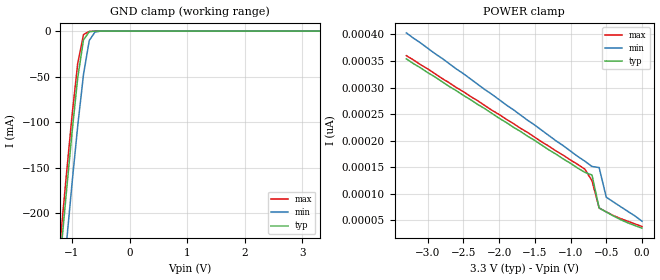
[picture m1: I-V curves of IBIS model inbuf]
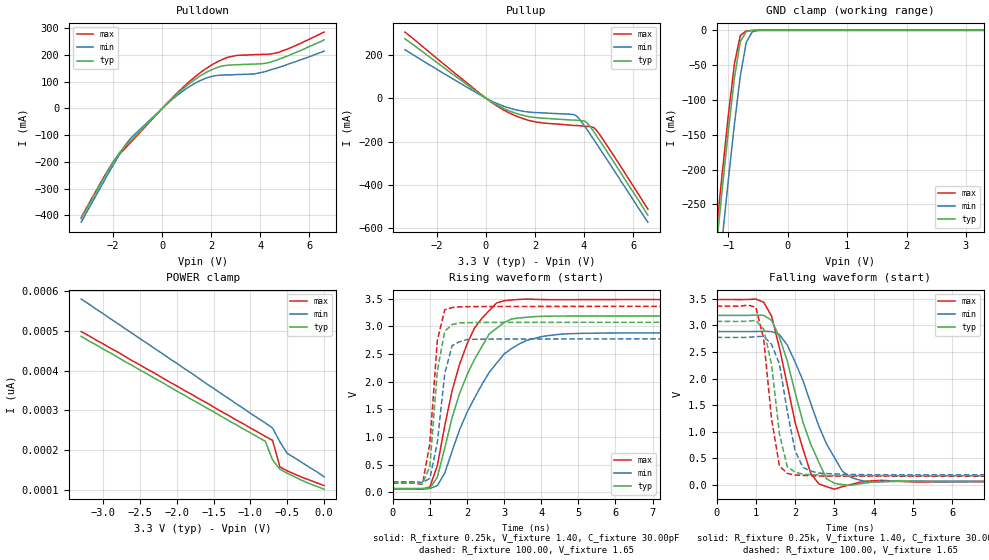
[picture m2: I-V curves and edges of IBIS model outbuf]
| IBIS file 163827.ibs created by s2ibis2 version 1.1
| North Carolina State University Electronics Research Laboratory  1995
[IBIS ver]   2.1
[File name]   163827.ibs
[File Rev]   1.0
[Date]   06/13/01
[Source]   Integrated Device Technology, Inc.
[Notes]   1.Temperatures: typ=25C, min=100C, max=0C 2.RRmp rates based
   on 50 ohm load.
[Disclaimer] Integrated Device Technology, Inc. ("IDT") hereby grants the
   user of this IBIS model a non-exclusive, nontransferable
   license to use this IBIS model under the following terms. The
   user is granted this license only to use the IBIS model and is
   not granted rights to sell, copy (except as needed to run the
   IBIS model), rent, lease or sub-license the IBIS model in
   whole or in part, or in modified form to anyone. The User may
   modify the IBIS model to suit its specific applications, but
   rights to derivative works and such modifications shall belong
   to IDT. This IBIS model is provided on an AS IS" basis and IDT
   makes absolutely no warranty with respect to the information
   contained herein. IDT DISCLAIMS AND CUSTOMER WAIVES ALL
   WARRANTIES, EXPRESS AND IMPLIED, INCLUDING WARRANTIES OF
   MERCHANTABILITY AND FITNESS FOR A PARTICULAR PURPOSE. THE
   ENTIRE RISK AS TO QUALITY AND PERFORMANCE IS WITH THE USER
   ACCORDINGLY, IN NO EVENT SHALL IDT BE LIABLE FOR ANY DIRECT OR
   INDIRECT DAMAGES, WHETHER IN CONTRACT OR TORT, INCLUDING ANY
   LOST PROFITS OR OTHER INCIDENTAL, CONSEQUENTIAL, EXEMPLARY, OR
   PUNITIVE DAMAGES ARISING OUT OF THE USE OR APPLICATION OF THE
   IBIS model. Further, IDT reserves the right to make changes
   without notice to any product herein to improve reliability,
   function, or design. IDT does not convey any license under
   patent rights or any other intellectual property rights,
   including those of third parties. IDT is not obligated to
   provide maintenance or support for the licensed IBIS model.
[Copyright]   Copyright 1997, Integrated Device Technology, Inc. all rights
   reserved
|   Component 74FCT163827A/B/C
[Component]   74FCT163827A/B/C
[Manufacturer]   Integrated Device Technology
[Package]
| PA56
| variable   typ   min   max
R_pkg   6.50m   5.00m   10.00m
L_pkg   3.30nH   2.50nH   4.90nH
C_pkg   0.29pF   0.010pF   1.16pF
[Pin]  signal_name   model_name   R_pin   L_pin   C_pin
1   1OE1_   inbuf
2   1Y1   outbuf
3   1Y2   outbuf
4   GND   GND
5   1Y3   outbuf
6   1Y4   outbuf
7   VCC   POWER
8   1Y5   outbuf
9   1Y6   outbuf
10   1Y7   outbuf
11   GND   GND
12   1Y8   outbuf
13   1Y9   outbuf
14   1Y10   outbuf
15   2Y1   outbuf
16   2Y2   outbuf
17   2Y3   outbuf
18   GND   GND
19   2Y4   outbuf
20   2Y5   outbuf
21   2Y6   outbuf
22   VCC   POWER
23   2Y7   outbuf
24   2Y8   outbuf
25   GND   GND
26   2Y9   outbuf
27   2Y10   outbuf
28   2OE1_   inbuf
29   2OE2_   inbuf
30   2A10   inbuf
31   2A9   inbuf
32   GND   GND
33   2A8   inbuf
34   2A7   inbuf
35   VCC   POWER
36   2A6   inbuf
37   2A5   inbuf
38   2A4   inbuf
39   GND   GND
40   2A3   inbuf
41   2A2   inbuf
42   2A1   inbuf
43   1A10   inbuf
44   1A9   inbuf
45   1A8   inbuf
46   GND   GND
47   1A7   inbuf
48   1A6   inbuf
49   1A5   inbuf
50   VCC   POWER
51   1A4   inbuf
52   1A3   inbuf
53   GND   GND
54   1A2   inbuf
55   1A1   inbuf
56   1OE2_   inbuf
| Models and submodels in the file (2): inbuf (Input), outbuf (3-state)
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| in   in   dummy_model
| oe   oe   dummy_model
|   Model inbuf
[Model]   inbuf
Model_type   Input
Vinl =  0.800V
Vinh =  2.000V
C_comp   3.00pF   NA   NA
[Temperature Range]   25.00   100.00   0.000
[Voltage Range]   3.30V   3.00V   3.60V
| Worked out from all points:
|   GND clamp passes 1 mA (typ) near -0.70 V on its own axis
[GND_clamp]
| voltage   I(typ)   I(min)   I(max)
-3.3V     -1.806A    -1.858A    -1.789A
-1.2V     -248mA     -306mA     -229mA
-1.1V     -179mA     -236mA     -160mA
-1V       -112mA     -168mA     -93.56mA
-900mV    -51.39mA   -104mA     -35.36mA
-800mV    -9.697mA   -47.7mA    -3.786mA
-700mV    -714uA     -10.4mA    -348uA
-600mV    -52.42uA   -951uA     -8.225uA
-500mV    -126nA     -30.48uA   -10.89nA
3.3V      34.69pA    75.27pA    23pA
[POWER_clamp]
| voltage   I(typ)   I(min)   I(max)
-3.3V     354pA      403pA      360pA
-800mV    140pA      161pA      146pA
-700mV    135pA      151pA      124pA
-600mV    72.75pA    149pA      72.79pA
-500mV    65.09pA    93.05pA    65.39pA
-300mV    50.77pA    75.27pA    52.78pA
0V        34.68pA    47.91pA    37.83pA
|   Model outbuf
[Model]   outbuf
Model_type   3-state
Polarity   Non-Inverting
Enable   Active-High
Vinl =  0.000V
Vinh =  2.000V
Vmeas =  1.500V
C_comp   3.00pF   NA   NA
[Temperature Range]   25.00   100.00   0.000
[Voltage Range]   3.30V   3.00V   3.60V
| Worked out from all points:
|   slope of the pulldown table from 0 to 0.495 V, typ, clamps not added: 11.1 ohm
|   slope of the pullup table from 0 to 0.495 V, typ, clamps not added: 14.5 ohm
|   GND clamp passes 1 mA (typ) near -0.65 V on its own axis
|   rising waveform, R_fixture 0.25k, V_fixture 1.40, C_fixture 30.00pF: 20-80 % time 982ps typ, 1.24ns min, 811ps max; typ from 0.061 V to 3.19 V
|   rising waveform, R_fixture 100.00, V_fixture 1.65: 20-80 % time 251ps typ, 304ps min, 220ps max; typ from 0.171 V to 3.08 V
|   falling waveform, R_fixture 0.25k, V_fixture 1.40, C_fixture 30.00pF: 20-80 % time 747ps typ, 915ps min, 646ps max; typ from 3.19 V to 0.061 V
|   falling waveform, R_fixture 100.00, V_fixture 1.65: 20-80 % time 336ps typ, 378ps min, 296ps max; typ from 3.08 V to 0.171 V
[Pulldown]
| voltage   I(typ)   I(min)   I(max)
-3.3V     -413mA     -426mA     -409mA
-2.1V     -217mA     -229mA     -215mA
-1.8V     -173mA     -182mA     -178mA
-1.4V     -132mA     -125mA     -139mA
100mV     9.36mA     8.53mA     9.88mA
900mV     77.5mA     68.6mA     83.2mA
1.8V      135mA      114mA      150mA
2.6V      161mA      126mA      189mA
3.7V      166mA      129mA      201mA
4.4V      173mA      144mA      204mA
5.1V      196mA      165mA      222mA
6.6V      257mA      215mA      286mA
[Pullup]
| voltage   I(typ)   I(min)   I(max)
-3.3V     273mA      223mA      304mA
-200mV    15.7mA     12.6mA     17.8mA
800mV     -51.2mA    -39.9mA    -59.2mA
1.4V      -75.9mA    -58mA      -89.7mA
2V        -89.2mA    -66.1mA    -109mA
3.5V      -101mA     -74.3mA    -125mA
3.7V      -102mA     -83mA      -126mA
4.1V      -112mA     -141mA     -130mA
4.4V      -155mA     -191mA     -136mA
4.5V      -172mA     -208mA     -147mA
5.2V      -292mA     -329mA     -263mA
6.6V      -539mA     -571mA     -511mA
[GND_clamp]
| voltage   I(typ)   I(min)   I(max)
-3.3V     -2.206A    -2.271A    -2.184A
-1.2V     -310mA     -382mA     -286mA
-1.1V     -225mA     -297mA     -202mA
-1V       -144mA     -214mA     -121mA
-900mV    -69.29mA   -136mA     -48.96mA
-800mV    -16.14mA   -65.88mA   -7.431mA
-700mV    -1.8mA     -17.54mA   -933uA
-600mV    -143uA     -2.267mA   -21.88uA
-500mV    -316nA     -75.99uA   -26.99nA
3.3V      101pA      168pA      89pA
[POWER_clamp]
| voltage   I(typ)   I(min)   I(max)
-3.3V     486pA      580pA      498pA
-800mV    222pA      268pA      234pA
-700mV    175pA      255pA      224pA
-600mV    151pA      220pA      157pA
-500mV    141pA      191pA      147pA
-300mV    123pA      168pA      131pA
0V        101pA      132pA      110pA
[Ramp]
| variable   typ   min   max
dV/dt_r   1.45/0.32n   1.21/0.34n   1.64/0.23n
dV/dt_f   1.59/0.39n   1.41/0.50n   1.76/0.35n
R_load = 50.00
[Rising Waveform]
R_fixture = 0.25k
V_fixture = 1.40
C_fixture = 30.00pF
R_dut = 7.00m
L_dut = 3.30nH
C_dut = 0.29pF
| time   V(typ)   V(min)   V(max)
0s        61.33mV    67.59mV    57.9mV
1ns       68.18mV    64.46mV    95.45mV
1.2ns     271mV      118mV      480mV
1.4ns     796mV      346mV      1.199V
1.6ns     1.353V     747mV      1.841V
2ns       2.123V     1.442V     2.681V
2.6ns     2.864V     2.17V      3.286V
3ns       3.069V     2.5V       3.464V
4.6ns     3.186V     2.863V     3.483V
19.8ns    3.189V     2.884V     3.487V
[Rising Waveform]
R_fixture = 100.00
V_fixture = 1.65
R_dut = 7.00m
L_dut = 3.30nH
C_dut = 0.29pF
| time   V(typ)   V(min)   V(max)
0s        171mV      188mV      162mV
600ps     171mV      189mV      159mV
800ps     145mV      174mV      142mV
1ns       470mV      249mV      885mV
1.2ns     2.193V     898mV      2.744V
1.4ns     2.912V     2.145V     3.3V
1.6ns     3.033V     2.652V     3.34V
2ns       3.067V     2.762V     3.356V
2.6ns     3.071V     2.77V      3.359V
19.8ns    3.075V     2.775V     3.362V
[Falling Waveform]
R_fixture = 0.25k
V_fixture = 1.40
C_fixture = 30.00pF
R_dut = 7.00m
L_dut = 3.30nH
C_dut = 0.29pF
| time   V(typ)   V(min)   V(max)
0s        3.189V     2.884V     3.487V
1ns       3.194V     2.885V     3.496V
1.4ns     3.097V     2.883V     3.176V
1.8ns     2.332V     2.631V     1.885V
2.4ns     759mV      1.527V     214mV
2.8ns     115mV      768mV      -35.65mV
3ns       29.9mV     514mV      -81.29mV
3.4ns     -10.27mV   148mV      3.984mV
4ns       54.08mV    51.85mV    76.18mV
19.8ns    61.33mV    67.6mV     57.91mV
[Falling Waveform]
R_fixture = 100.00
V_fixture = 1.65
R_dut = 7.00m
L_dut = 3.30nH
C_dut = 0.29pF
| time   V(typ)   V(min)   V(max)
0s        3.075V     2.775V     3.362V
1ns       3.095V     2.788V     3.342V
1.2ns     2.928V     2.795V     2.746V
1.4ns     2.266V     2.644V     1.244V
1.6ns     960mV      2.279V     356mV
1.8ns     340mV      1.382V     216mV
2ns       239mV      641mV      185mV
2.2ns     199mV      327mV      178mV
2.6ns     183mV      221mV      166mV
19.8ns    171mV      188mV      162mV
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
